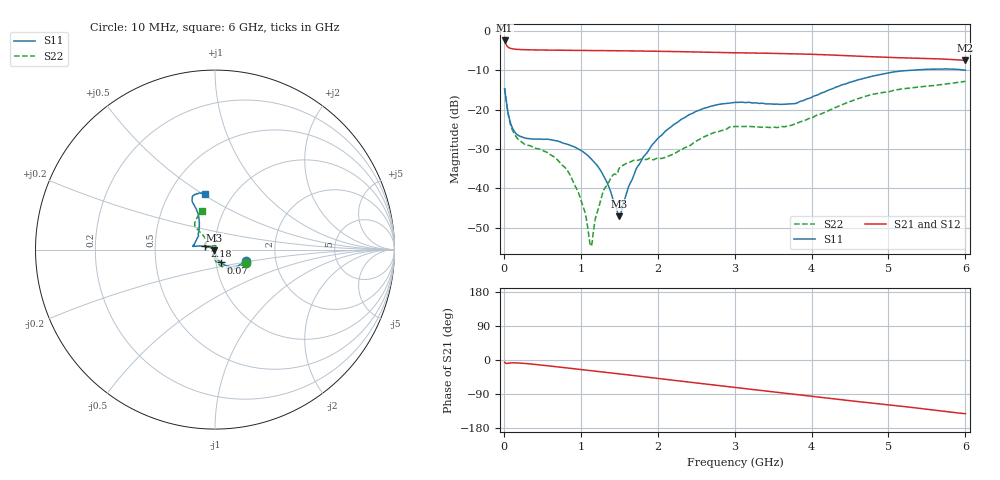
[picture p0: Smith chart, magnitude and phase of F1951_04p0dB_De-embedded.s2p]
! Integrated Device Technology
! Corporate Headquarters
! 6024 Silver Creek Valley Road
! San Jose, CA 95138  USA
! Phone:  1-408-284-8200
! Toll Free:  1-800-223-1366
! Webpage:  http://www.idt.com/
! Timing and RF Division
! 515 Groton Road, Suite 102
! Westford, MA 01886-6024
! Device:  F1951
! Description: 6-bit 0.5 dB Digital Step Attenuator
! Frequency:  100.0 -  4000.00 MHz
! Package:  4x4 mm Thin QFN Plastic Package: 24 pin
! Ports:  2 RF, 6 DC
!  Pin  1  = NC
!  Pin  2  = RF1  =  Port 1
!  Pin  3  = GND
!  Pin  4  = NC
!  Pin  5  = Serial Data Out (SDO)
!  Pin  6  = NC
!  Pin  7  = Reset Bar ( RSTb)
!  Pin  8  = Clock (CLK)
!  Pin  9  = Chip Select Bar (CSb)
!  Pin 10  = NC
!  Pin 11  = Serial Data In (SDI)
!  Pin 12  = NC
!  Pin 13  = NC
!  Pin 14  = VDD
!  Pin 15  = NC
!  Pin 16  = GND
!  Pin 17  = RF2  =  Port 2
!  Pin 18  = NC
!  Pin 19  = GND
!  Pin 20  = GND
!  Pin 21  = GND
!  Pin 22  = GND
!  Pin 23  = GND
!  Pin 24  = GND
! State:  8
! Atten State:  4.0 dB
! Voltage:  +3.30 Volts
! Current:  0.475 mA
! Data:  The device was measured on a F195X evaluation board which has
!  individual transmission lines to the RF pins.  Data was collected
!  de-embedded using a Automatic Fixture Removal [AFR] (Keysight Technologies).
!  The reference plane is the edge of the package pin.
! Misc:  Lot Code  1225BCA
!  Action Tracker AT0399
! Date Measured:  2018-09-13
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# GHz S dB R 50
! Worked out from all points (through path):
!   600 points, 10 MHz to 6 GHz, reference 50 ohm
!   highest |S21| = -2.43 dB at 10 MHz (marker M1); lowest = -7.5 dB at 6 GHz (marker M2)
!   group delay of S21, straight-line fit = 64.5 ps
!   lowest |S11| = -47.1 dB at 1.5 GHz (marker M3), VSWR 1.01, Z = 49.7 - j0.297 ohm
!   |S11| at or under -10 dB: start of sweep to 5.317 GHz
!   |S22| runs from -54.7 to -12.8 dB; largest |S21 - S12| = 0.00073
!   S11 on the Smith chart (normalised r, x): 10 MHz: 1.40, -0.19; 70 MHz: 1.05, -0.15; 2.18 GHz: 0.89, +0.03; 6 GHz: 0.74, +0.51
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0.01  -14.75 -21.2  -2.43 -5.4  -2.43 -5.4  -14.56 -23.6
0.07  -22.18 -66.5  -4.32 -8.0  -4.32 -8.1  -22.53 -80.3
0.13  -25.37 -77.2  -4.61 -7.4  -4.61 -7.4  -25.96 -96.4
0.21  -26.78 -84.6  -4.73 -8.1  -4.73 -8.1  -27.92 -106.8
0.57  -27.55 -90.2  -4.88 -15.2  -4.88 -15.2  -30.99 -114.5
0.8  -28.65 -85.7  -4.93 -20.4  -4.93 -20.4  -34.83 -110.7
1.01  -30.46 -79.8  -4.98 -25.2  -4.98 -25.2  -43.49 -93.3
1.06  -31.14 -80.2  -4.99 -26.4  -4.99 -26.3  -46.52 -82.1
1.11  -32.03 -79.6  -4.99 -27.4  -4.99 -27.4  -52.80 -44.0
1.14  -32.63 -79.8  -5.00 -28.1  -5.00 -28.1  -54.66 -8.8
1.21  -34.14 -80.5  -5.00 -29.8  -5.01 -29.8  -46.34 53.0
1.3  -37.01 -82.6  -5.01 -31.9  -5.02 -31.9  -40.39 63.6
1.5  -47.11 -137.3  -5.07 -36.5  -5.07 -36.5  -34.95 78.7
1.73  -34.75 155.8  -5.11 -42.1  -5.11 -42.1  -32.89 85.9
2.01  -27.18 159.3  -5.19 -48.8  -5.19 -48.8  -32.33 110.3
2.18  -24.28 162.1  -5.24 -52.8  -5.24 -52.9  -31.48 130.7
2.58  -19.82 168.9  -5.38 -62.5  -5.39 -62.4  -27.13 163.3
3.01  -18.16 171.6  -5.55 -72.5  -5.56 -72.4  -24.30 167.9
3.65  -18.61 149.1  -5.77 -87.6  -5.77 -87.5  -24.36 143.4
4.01  -16.78 127.5  -5.95 -96.1  -5.95 -96.1  -22.04 131.4
5.01  -10.66 115.4  -6.75 -118.6  -6.75 -118.6  -15.44 130.3
6  -9.97 100.5  -7.49 -141.7  -7.49 -141.7  -12.83 108.7
